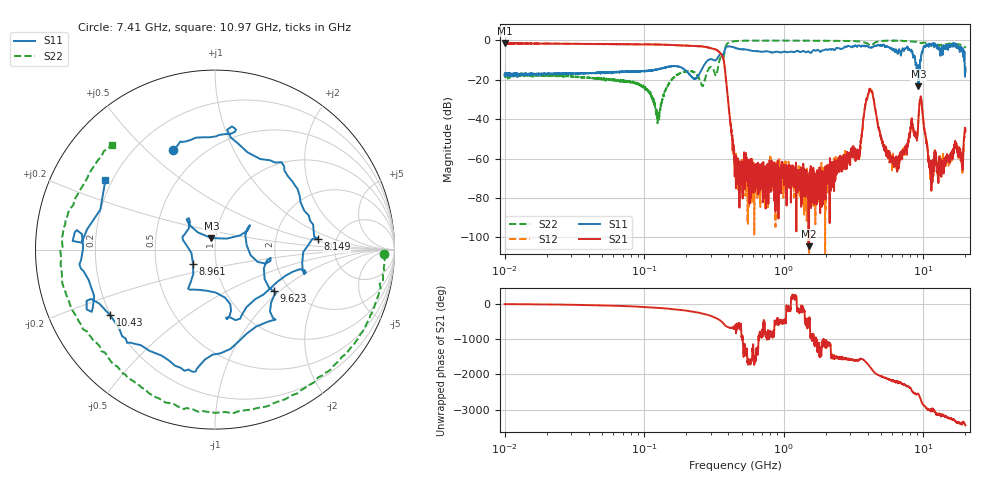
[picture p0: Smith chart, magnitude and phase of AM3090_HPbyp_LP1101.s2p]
# Hz S DB R 50
!freq MagS11 AngS11 MagS21 AngS21 MagS12 AngS12 MagS22 AngS22
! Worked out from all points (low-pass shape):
!   3201 points, 10 MHz to 20 GHz, reference 50 ohm
!   highest |S21| = -1.46 dB at 10.05 MHz (marker M1); lowest = -104.4 dB at 1.505 GHz (marker M2)
!   |S21| within 3 dB of the highest: start of sweep to 314.8 MHz
!   lowest |S11| = -23.5 dB at 9.22 GHz (marker M3), VSWR 1.14, Z = 47.6 + j6.12 ohm
!   |S11| at or under -10 dB: start of sweep to 289 MHz; 8.729 GHz to 9.574 GHz (844.2 MHz wide, 9.22 % of centre); 19.73 GHz to end of sweep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
!   |S22| runs from -42.1 to -0.2 dB; largest |S21 - S12| = 0.033
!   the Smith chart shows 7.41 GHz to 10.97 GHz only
!   S11 on the Smith chart (normalised r, x): 7.41 GHz: 0.35, +0.61; 8.149 GHz: 3.58, +0.63; 8.961 GHz: 0.77, -0.13; 9.623 GHz: 1.66, -0.92; 10.43 GHz: 0.20, -0.28; 10.97 GHz: 0.17, +0.28
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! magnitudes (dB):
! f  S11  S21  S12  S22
! 10 MHz  -17.6  -1.6  -1.6  -16.9
! 10.05 MHz  -17.2  -1.5  -1.7  -18.6
! 35.55 MHz  -16.8  -1.9  -1.9  -18.7
! 93.92 MHz  -16.0  -2.1  -2.1  -23.3
! 126.1 MHz  -14.8  -2.2  -2.2  -38.4
! 165.3 MHz  -13.1  -2.5  -2.5  -18.6
! 354.3 MHz  -7.1  -7.0  -6.9  -8.6
! 447.2 MHz  -3.9  -61.1  -60.6  -0.5
! 1.505 GHz  -5.8  -104.4  -77.6  -0.3
! 1.59 GHz  -5.9  -73.3  -68.3  -0.2
! 3.424 GHz  -2.7  -57.5  -56.1  -0.7
! 4.141 GHz  -3.8  -25.3  -25.8  -2.6
! 5.639 GHz  -3.6  -58.5  -59.4  -0.3
! 7.41 GHz  -4.4  -53.9  -54.9  -0.5
! 8.149 GHz  -4.8  -41.9  -44.1  -0.7
! 8.961 GHz  -16.7  -48.9  -50.0  -0.9
! 9.22 GHz  -23.5  -39.4  -39.5  -1.1
! 9.623 GHz  -7.9  -29.6  -29.5  -1.5
! 10.43 GHz  -3.2  -49.4  -49.8  -1.4
! 10.97 GHz  -2.8  -61.1  -59.1  -1.7
! 18.67 GHz  -3.6  -58.3  -58.7  -2.4
! 20 GHz  -13.9  -46.4  -44.9  -4.0
